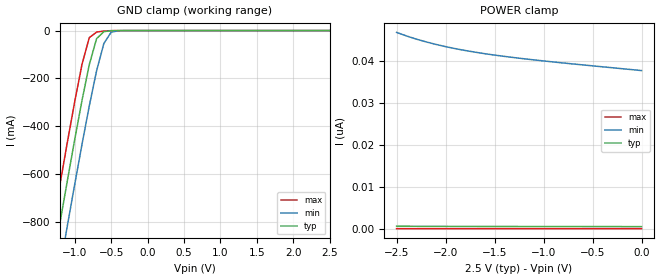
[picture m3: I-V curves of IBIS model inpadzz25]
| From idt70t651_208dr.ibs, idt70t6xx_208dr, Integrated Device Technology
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|   Model inpadzz25
[Model]   inpadzz25
Model_type   Input
Polarity   Non-Inverting
Vinl =  0.80000V
Vinh =  2.00000V
Vmeas =  1.50000V
C_comp   4.50000pF   4.50000pF   4.50000pF
[Temperature Range]   25.00000   100.00000   -40.00000
[Voltage Range]   2.50000V   2.20000V   2.80000V
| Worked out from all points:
|   GND clamp passes 1 mA (typ) near -0.51 V on its own axis
[GND_clamp]
| voltage   I(typ)   I(min)   I(max)
-2.5V     -3.145A    -3.326A    -2.992A
-1.4V     -1.152A    -1.34A     -992.6mA
-1.3V     -975mA     -1.163A    -814.5mA
-1.2V     -799.1mA   -987.7mA   -638.3mA
-1.1V     -625.5mA   -813.9mA   -465mA
-900mV    -292mA     -475.5mA   -141.4mA
-800mV    -142.5mA   -315.2mA   -29.66mA
-700mV    -33.97mA   -168.4mA   -6.415mA
-600mV    -4.291mA   -54.25mA   -1.765mA
-500mV    -767.5uA   -6.912mA   -190.3uA
-400mV    -75.7uA    -637.7uA   -8.282uA
2.5V      493.9pA    38.32nA    3.386pA
[POWER_clamp]
| voltage   I(typ)   I(min)   I(max)
-2.5V     588.9pA    46.73nA    4.616pA
-2.4V     578.8pA    45.89nA    4.553pA
-2.3V     569.9pA    45.14nA    4.503pA
-2.2V     562pA      44.48nA    4.452pA
-2.1V     555pA      43.88nA    4.404pA
-1.9V     543.3pA    42.86nA    4.294pA
-1.8V     538.5pA    42.42nA    4.255pA
-1.6V     530.2pA    41.66nA    4.162pA
-1.4V     523.5pA    41.02nA    4.079pA
-1.1V     515.4pA    40.19nA    3.956pA
-800mV    508.8pA    39.45nA    3.825pA
0V        493.9pA    37.64nA    3.507pA
